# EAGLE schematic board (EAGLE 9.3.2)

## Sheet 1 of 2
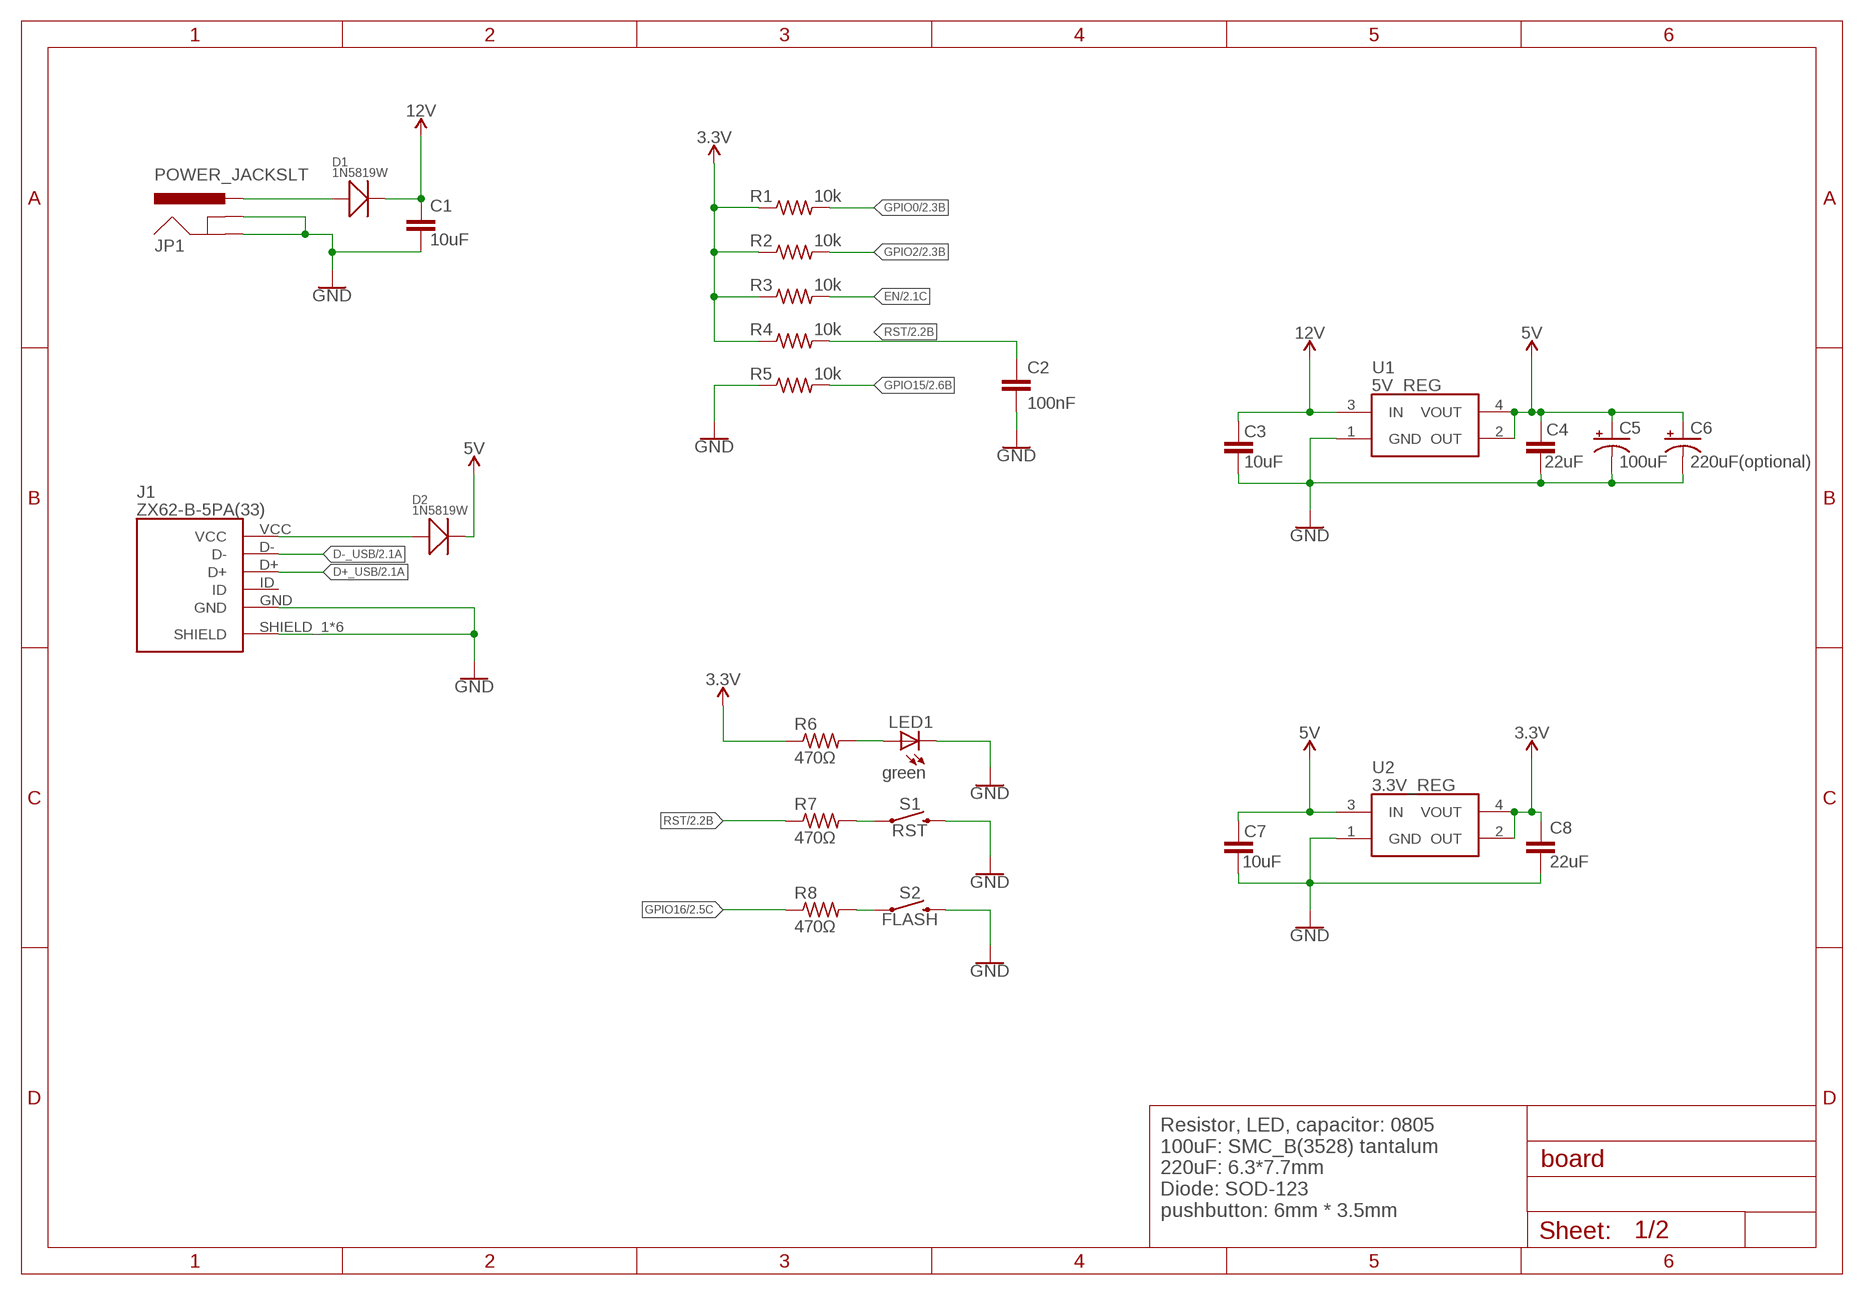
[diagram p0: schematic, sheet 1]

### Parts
C1  10uF  C-EUC0805  [C0805]
C2  100nF  C-EUC0805  [C0805]
C3  10uF  C-EUC0805  [C0805]
C4  22uF  C-EUC0805  [C0805]
C5  100uF  CPOL-USSMCB  [SMC_B]
C6  220uF(optional)  CPOL-USUD-6,3X7,7  [UD-6,3X7,7_NICHICON]
C7  10uF  C-EUC0805  [C0805]
C8  22uF  C-EUC0805  [C0805]
D1  1N5819W  SMD-DIODE-SCHOTTKY-20V-500MA(SOD-123)  [SOD-123]
D2  1N5819W  SMD-DIODE-SCHOTTKY-20V-500MA(SOD-123)  [SOD-123]
J1  ZX62-B-5PA(33)  [ZX62B5PA33]
JP1  POWER_JACKSLT  [POWER_JACK_SLOT]
LED1  green  LEDCHIP-LED0805  [CHIP-LED0805]
R1  10k  R-US_R0805  [R0805]
R2  10k  R-US_R0805  [R0805]
R3  10k  R-US_R0805  [R0805]
R4  10k  R-US_R0805  [R0805]
R5  10k  R-US_R0805  [R0805]
R6  470Ω  R-US_R0805  [R0805]
R7  470Ω  R-US_R0805  [R0805]
R8  470Ω  R-US_R0805  [R0805]
S1  RST  MOMENTARY-SWITCH-SPST-SMD-6.0X3.5MM  [TACTILE_SWITCH_SMD_6.0X3.5MM]
S2  FLASH  MOMENTARY-SWITCH-SPST-SMD-6.0X3.5MM  [TACTILE_SWITCH_SMD_6.0X3.5MM]
U1  5V_REG  AZ1117H-5.0TRE1  [SOT230P700X170-4N]
U2  3.3V_REG  AZ1117H-5.0TRE1  [SOT230P700X170-4N]

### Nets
3.3V [power]: C8.2 R1.1 R2.1 R3.1 R4.1 R6.1 U2.2(OUT) U2.4(VOUT) ; also sheet 2
5V [power]: C4.1 C5.+ C6.+ C7.1 D2.- U1.2(OUT) U1.4(VOUT) U2.3(IN) ; also sheet 2
5V_INPUT [power]: D2.+ J1.VCC
12V [power]: C1.2 C3.1 D1.- U1.3(IN) ; also sheet 2
12V_INPUT [power]: D1.+ JP1.PWR
D+_USB: J1.D+ ; also sheet 2
D-_USB: J1.D- ; also sheet 2
EN: R3.2 ; also sheet 2
GND [power]: C1.1 C2.1 C3.2 C4.2 C5.- C6.- C7.2 C8.1 J1.GND J1.SHIELD_1(SHIELD) J1.SHIELD_2(SHIELD) J1.SHIELD_3(SHIELD) J1.SHIELD_4(SHIELD) J1.SHIELD_5(SHIELD) J1.SHIELD_6(SHIELD) JP1.GND@1(GNDBREAK) JP1.GND@2(GND) LED1.C R5.1 S1.2 S2.2 U1.1(GND) U2.1(GND) ; also sheet 2
GPIO0: R1.2 ; also sheet 2
GPIO2: R2.2 ; also sheet 2
GPIO15: R5.2 ; also sheet 2
GPIO16: R8.1 ; also sheet 2
N$4: LED1.A R6.2
POWER: R7.2 S1.1
POWER1: R8.2 S2.1
RST: C2.2 R4.2 R7.1 ; also sheet 2
Unconnected: J1.ID

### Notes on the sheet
- Resistor, LED, capacitor: 0805
  100uF: SMC_B(3528) tantalum
  220uF: 6.3*7.7mm
  Diode: SOD-123
  pushbutton: 6mm * 3.5mm

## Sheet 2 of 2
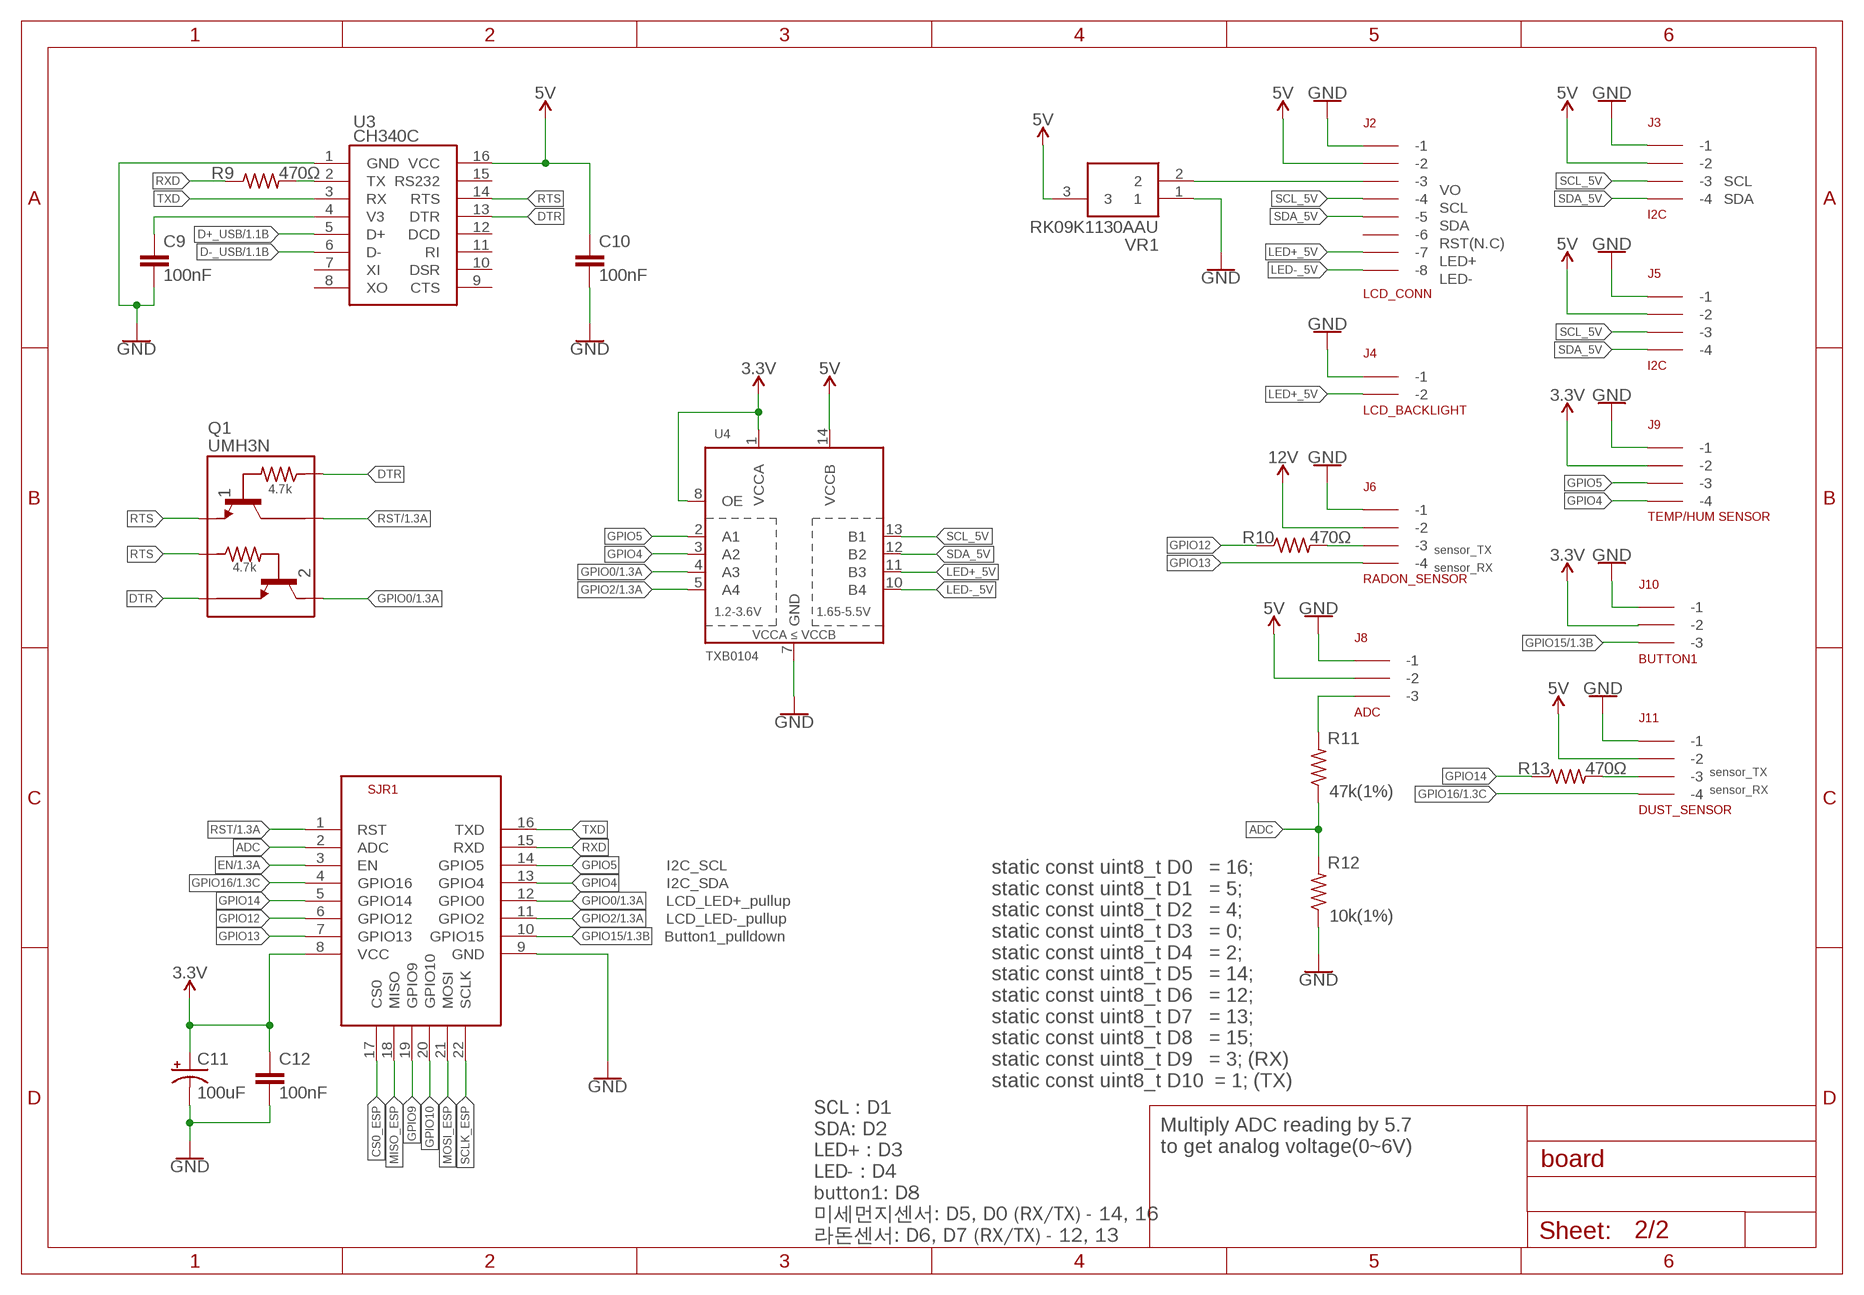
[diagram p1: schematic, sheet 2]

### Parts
C9  100nF  C-EUC0805  [C0805]
C10  100nF  C-EUC0805  [C0805]
C11  100uF  CPOL-USSMCB  [SMC_B]
C12  100nF  C-EUC0805  [C0805]
J2  LCD_CONN  5267-8  [5267-8]
J3  I2C  5267-4  [5267-4]
J4  LCD_BACKLIGHT  5267-2  [5267-2]
J5  I2C  5267-4  [5267-4]
J6  RADON_SENSOR  5267-4  [5267-4]
J8  ADC  5267-3  [5267-3]
J9  TEMP/HUM SENSOR  5267-4  [5267-4]
J10  BUTTON1  5267-3  [5267-3]
J11  DUST_SENSOR  5267-4  [5267-4]
Q1  UMH3N  UMH3NFHATN  [SOT65P210X100-6N]
R9  470Ω  R-US_R0805  [R0805]
R10  470Ω  R-US_R0805  [R0805]
R11  47k(1%)  R-US_R0805  [R0805]
R12  10k(1%)  R-US_R0805  [R0805]
R13  470Ω  R-US_R0805  [R0805]
SJR1  ESP-12E  ESP8266-12EESP12E  [ESP8266-ESP12E]
U3  CH340C  CH340G  [SOIC16]
U4  TXB0104  TXB0104PWR  [TSSOP14]
VR1  RK09K1130AAU  RK09K1130A6S  [RK09K1130BGM]

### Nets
3.3V [power]: C11.+ C12.2 J9.P$2(-2) J10.P$2(-2) SJR1.8(VCC) U4.1(VCCA) U4.8(OE) ; also sheet 1
5V [power]: C10.2 J2.P$2(-2) J3.P$2(-2) J5.P$2(-2) J8.P$2(-2) J11.P$2(-2) U3.16(VCC) U4.14(VCCB) VR1.3 ; also sheet 1
12V [power]: J6.P$2(-2) ; also sheet 1
ADC: R11.1 R12.2 SJR1.2(ADC)
CS0_ESP: SJR1.17(CS0)
D+_USB: U3.5(D+) ; also sheet 1
D-_USB: U3.6(D-) ; also sheet 1
DTR: Q1.2 Q1.4 U3.13(DTR)
EN: SJR1.3(EN) ; also sheet 1
GND [power]: C9.1 C10.1 C11.- C12.1 J2.P$1(-1) J3.P$1(-1) J4.P$1(-1) J5.P$1(-1) J6.P$1(-1) J8.P$1(-1) J9.P$1(-1) J10.P$1(-1) J11.P$1(-1) R12.1 SJR1.9(GND) U3.1(GND) U4.7(GND) VR1.1 ; also sheet 1
GPIO0: Q1.3 SJR1.12(GPIO0) U4.4(A3) ; also sheet 1
GPIO2: SJR1.11(GPIO2) U4.5(A4) ; also sheet 1
GPIO4: J9.P$4(-4) SJR1.13(GPIO4) U4.3(A2)
GPIO5: J9.P$3(-3) SJR1.14(GPIO5) U4.2(A1)
GPIO9: SJR1.19(GPIO9)
GPIO10: SJR1.20(GPIO10)
GPIO12: R10.1 SJR1.6(GPIO12)
GPIO13: J6.P$4(-4) SJR1.7(GPIO13)
GPIO14: R13.1 SJR1.5(GPIO14)
GPIO15: J10.P$3(-3) SJR1.10(GPIO15) ; also sheet 1
GPIO16: J11.P$4(-4) SJR1.4(GPIO16) ; also sheet 1
LED+_5V: J2.P$7(-7) J4.P$2(-2) U4.11(B3)
LED-_5V: J2.P$8(-8) U4.10(B4)
MISO_ESP: SJR1.18(MISO)
MOSI_ESP: SJR1.21(MOSI)
N$1: C9.2 U3.4(V3)
N$2: J2.P$3(-3) VR1.2
N$3: R9.2 U3.2(TX)
N$5: J8.P$3(-3) R11.2
N$6: J6.P$3(-3) R10.2
N$9: J11.P$3(-3) R13.2
RST: Q1.6 SJR1.1(RST) ; also sheet 1
RTS: Q1.1 Q1.5 U3.14(RTS)
RXD: R9.1 SJR1.15(RXD)
SCL_5V: J2.P$4(-4) J3.P$3(-3) J5.P$3(-3) U4.13(B1)
SCLK_ESP: SJR1.22(SCLK)
SDA_5V: J2.P$5(-5) J3.P$4(-4) J5.P$4(-4) U4.12(B2)
TXD: SJR1.16(TXD) U3.3(RX)
Unconnected: J2.P$6(-6) U3.7(XI) U3.8(XO) U3.9(CTS) U3.10(DSR) U3.11(RI) U3.12(DCD) U3.15(RS232)

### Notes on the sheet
- SCL
- VO
- SDA
- SCL
- SDA
- RST(N.C)
- LED+
- LED-
- sensor_TX
- sensor_RX
- sensor_TX
- sensor_RX
- static const uint8_t D0   = 16;
  static const uint8_t D1   = 5;
  static const uint8_t D2   = 4;
  static const uint8_t D3   = 0;
  static const uint8_t D4   = 2;
  static const uint8_t D5   = 14;
  static const uint8_t D6   = 12;
  static const uint8_t D7   = 13;
  static const uint8_t D8   = 15;
  static const uint8_t D9   = 3; (RX)
  static const uint8_t D10  = 1; (TX)
- I2C_SCL
- I2C_SDA
- LCD_LED+_pullup
- LCD_LED-_pullup
- Button1_pulldown
- SCL : D1
  SDA: D2
  LED+ : D3
  LED- : D4
  button1: D8
  미세먼지센서: D5, D0 (RX/TX) - 14, 16
  라돈센서: D6, D7 (RX/TX) - 12, 13
- Multiply ADC reading by 5.7
  to get analog voltage(0~6V)

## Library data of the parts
C1-C4 C7-C10 C12 = rcl:C-EU: CAPACITOR, European symbol; SPICEPREFIX: C
C5 C6 C11 = rcl:CPOL-US: POLARIZED CAPACITOR, American symbol; SPICEPREFIX: C
D1 D2 = Seeed-Diode:SMD-DIODE-SCHOTTKY-20V-500MA(SOD-123): 304020032; MPN: SS0520-7-F; VALUE: 20V-500MA
J1 = SamacSys_Parts:ZX62-B-5PA(33): USB Connectors MICRO B RECEPT RA SMT BTTM MNT Source: Datasheet; DESCRIPTION: USB Connectors MICRO B RECEPT RA SMT BTTM MNT; HEIGHT: 2.8mm; MANUFACTURER_NAME: Hirose; MANUFACTURER_PART_NUMBER: ZX62-B-5PA(33); MOUSER_PART_NUMBER: 798-ZX62-B-5PA33; MOUSER_PRICE-STOCK: https://www.mouser.com/Search/Refine.aspx?Keyword=798-ZX62-B-5PA33
J2 = con-molex-spox:5267-8
J3 J5 J6 J9 J11 = con-molex-spox:5267-4
J4 = con-molex-spox:5267-2
J8 J10 = con-molex-spox:5267-3
JP1 = kanflo:POWER_JACK: Power Jack This is the standard 5.5mm barrel jack for power. The SLT footprint has been proven in designs produced by DirtyPCBs.com and only works if the mill layer is transmitted to the PCB fab house and the fab house accepts it. Rumours has it OSH Park accepts this design too. This symbol is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
LED1 = adafruit:LED: LED
Q1 = SamacSys_Parts:UMH3NFHATN: ROHM - UMH3NFHATN - TRANS, NPN, AUTO, 4.7K/4.7K, SOT-353 Source: Datasheet; DESCRIPTION: ROHM - UMH3NFHATN - TRANS, NPN, AUTO, 4.7K/4.7K, SOT-353; HEIGHT: 1mm; MANUFACTURER_NAME: ROHM Semiconductor; MANUFACTURER_PART_NUMBER: UMH3NFHATN; MOUSER_PART_NUMBER: 755-UMH3NFHATN; MOUSER_PRICE-STOCK: https://www.mouser.com/Search/Refine.aspx?Keyword=755-UMH3NFHATN
R1-R13 = rcl:R-US_: RESISTOR, American symbol; SPICEPREFIX: R
S1 S2 = SparkFun-Switches:MOMENTARY-SWITCH-SPST: Momentary Switch (Pushbutton) - SPST; PROD_ID: SWCH-00815; SF_SKU: COM-08229
SJR1 = esp12e:ESP8266-12E: ESP8266-12E Library for Eagle CAD The author not responsible for any damages or errors!. Created by Suhail jr.lt;/author>
U1 U2 = SamacSys_Parts:AZ1117H-5.0TRE1: 1A 5V LDO Linear Voltage Reg SOT-223 Diodes Inc AZ1117H-5.0TRE1, Single Linear Voltage Regulator, 1A 4.9 5.1 V, 1%, 3-Pin SOT-223 Source: Datasheet; DESCRIPTION: 1A 5V LDO Linear Voltage Reg SOT-223 Diodes Inc AZ1117H-5.0TRE1, Single Linear Voltage Regulator, 1A 4.9 5.1 V, 1%, 3-Pin SOT-223; HEIGHT: 1.7mm; MANUFACTURER_NAME: Diodes Inc.; MANUFACTURER_PART_NUMBER: AZ1117H-5.0TRE1; MOUSER_PART_NUMBER: 621-AZ1117H-5.0TRE1; MOUSER_PRICE-STOCK: https://www.mouser.com/Search/Refine.aspx?Keyword=621-AZ1117H-5.0TRE1
U3 = ch340g:CH340G
U4 = SparkFun-IC-Comms:TXB0104PWR: 4-Bit Bi-Directional Level Shifter 1.2V-3.6V (VCCA) to 1.65V-5.5V (VCCB) bi-directional level shifter with auto direction sensing. Max data rate - VCCA 1.8V: 20Mbps (50ns), VCCA 3.3V: 100Mbps (10ns) Digikey: 296-21929-1-ND (TSSOP) Datasheet SparkFun Products SparkFun Cellular Shield - MG2639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; PROD_ID: NA-XXXXX
VR1 = SamacSys_Parts:RK09K1130A6S: Audio single pot. 10K Vertical 15mm,1B Alps RK09K Series, Linear Potentiometer with a 6 mm Dia. Shaft, 10k, +/-20%, Through Hole Source: Datasheet; DESCRIPTION: Audio single pot. 10K Vertical 15mm,1B Alps RK09K Series, Linear Potentiometer with a 6 mm Dia. Shaft, 10k, +/-20%, Through Hole; HEIGHT: mm; MANUFACTURER_NAME: ALPS; MANUFACTURER_PART_NUMBER: RK09K1130A6S; MOUSER_PART_NUMBER: 688-RK09K1130A6S; MOUSER_PRICE-STOCK: https://www.mouser.com/Search/Refine.aspx?Keyword=688-RK09K1130A6S

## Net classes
0 default: width 0.203 mm
1 power: width 0.762 mm

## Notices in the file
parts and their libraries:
SparkFun-PowerSymbols: Licensing: Creative Commons ShareAlike 4.0 International - https://creativecommons.org/licenses/by-sa/4.0
